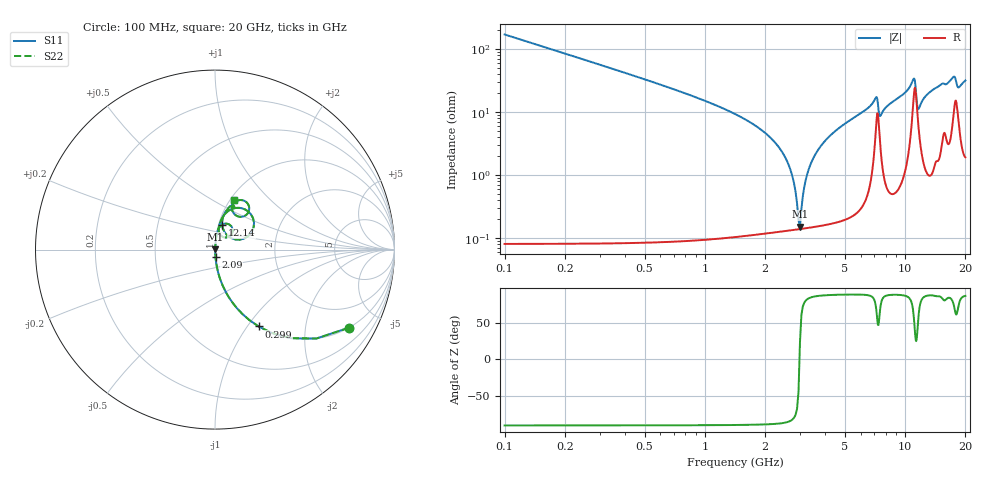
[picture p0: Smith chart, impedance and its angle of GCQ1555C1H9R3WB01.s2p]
!Murata Part Number: GCQ1555C1H9R3WB01
!These Parameters are Measured in Series Mode Connection
!Data Generated on Jan 08, 2026
!  o--ll--o
!Port1  Port2
!  o------o
!Operation Temp=25[degC], DC Bias Voltage=0[V]
!Freq. Start=100[MHz] Stop=20[GHz] 401[Steps]
# Hz S RI R 50
!Freq.(Hz) S11(Real) S11(Imag) S21(Real) S21(Imag) S12(Real) S12(Imag) S22(Real) S22(Imag)
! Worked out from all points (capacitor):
!   401 points, 100 MHz to 20 GHz, reference 50 ohm
!   read as one part in series: C = 9.3 pF near 199.5 MHz
!   lowest |Z| = 153 mohm at 2.986 GHz (marker M1)
!   series resonance near 2.97 GHz, so ESL is about 310 pH
!   S11 on the Smith chart (normalised r, x): 100 MHz: 1.00, -3.42; 299 MHz: 1.00, -1.13; 2.09 GHz: 1.00, -0.08; 12.14 GHz: 1.04, +0.29; 20 GHz: 1.04, +0.64
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1e8  0.7449 -0.4357  0.2551 0.4357  0.2551 0.4357  0.7449 -0.4357
2.99e8  0.2433 -0.4284  0.7567 0.4284  0.7567 0.4284  0.2433 -0.4284
7.4675e8  0.0448 -0.2049  0.9552 0.2049  0.9552 0.2049  0.0448 -0.2049
2.09e9  0.00291 -0.0413  0.9971 0.0413  0.9971 0.0413  0.00291 -0.0413
2.5875e9  0.00157 -0.016  0.9984 0.016  0.9984 0.016  0.00157 -0.016
2.73675e9  0.00143 -0.00947  0.9986 0.00947  0.9986 0.00947  0.00143 -0.00947
2.886e9  0.00139 -0.00332  0.9986 0.00332  0.9986 0.00332  0.00139 -0.00332
2.9855e9  0.0014 0.00061  0.9986 -0.00061  0.9986 -0.00061  0.0014 0.00061
3.23425e9  0.00155 0.00992  0.9985 -0.00992  0.9985 -0.00992  0.00155 0.00992
3.43325e9  0.00178 0.0169  0.9982 -0.0169  0.9982 -0.0169  0.00178 0.0169
4.42825e9  0.00408 0.0483  0.9959 -0.0483  0.9959 -0.0483  0.00408 0.0483
6.7665e9  0.0249 0.1255  0.9751 -0.1255  0.9751 -0.1255  0.0249 0.1255
7.1645e9  0.0782 0.1409  0.9218 -0.1409  0.9218 -0.1409  0.0782 0.1409
7.51275e9  0.0354 0.0762  0.9646 -0.0762  0.9646 -0.0762  0.0354 0.0762
1.005e10  0.052 0.1941  0.948 -0.1941  0.948 -0.1941  0.052 0.1941
1.099525e10  0.1837 0.2136  0.8163 -0.2136  0.8163 -0.2136  0.1837 0.2136
1.159225e10  0.0746 0.0741  0.9254 -0.0741  0.9254 -0.0741  0.0746 0.0741
1.21395e10  0.0401 0.1383  0.9599 -0.1383  0.9599 -0.1383  0.0401 0.1383
1.338325e10  0.0514 0.1987  0.9486 -0.1987  0.9486 -0.1987  0.0514 0.1987
1.67165e10  0.1128 0.2663  0.8872 -0.2663  0.8872 -0.2663  0.1128 0.2663
1.8408e10  0.1156 0.1914  0.8844 -0.1914  0.8844 -0.1914  0.1156 0.1914
2e10  0.1057 0.2788  0.8943 -0.2788  0.8943 -0.2788  0.1057 0.2788
